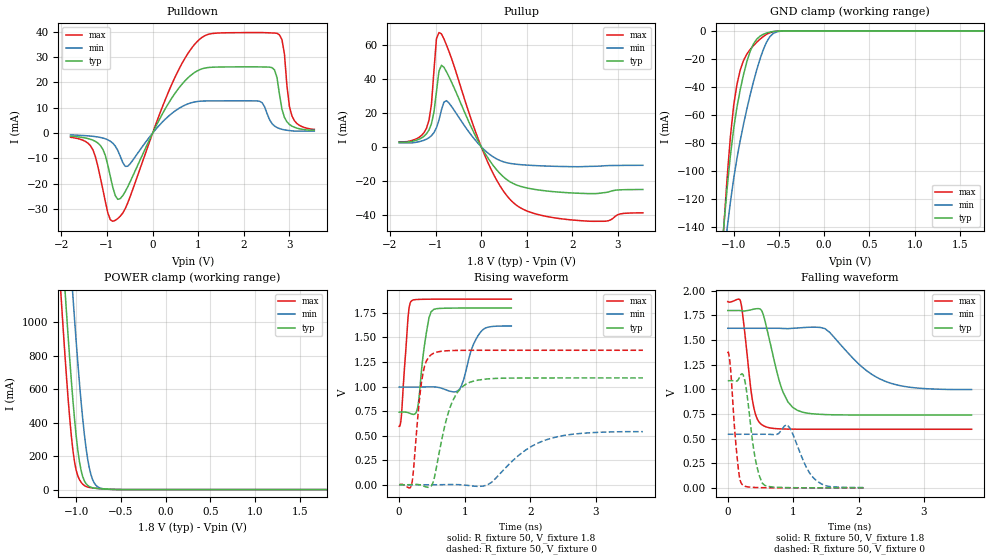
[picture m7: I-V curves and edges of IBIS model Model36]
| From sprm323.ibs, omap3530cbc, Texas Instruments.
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| Model based on original model for BQOMAPPROGIOCSHYFBPB_7LM
|   Sub model MODE10_PU_PD_OFF_1P8
[model]   Model36
|[Input Load]   PI
|[Output Drive] DS10
|Voltage   1.8V
|Mode   I/O
Model_type   I/O
Polarity   Non-Inverting
Enable   Active-Low
Vinl =  0.63
Vinh =  1.17
Cref =  15.0000pF
Rref =  100.0000M
Vref =  0V
Vmeas =  0.9
C_comp   0.8864943p   0.7714798p   1.034566p
[Model Spec]
Vinl   0.63   0.567   0.6615
Vinh   1.17   1.053   1.2285
[Temperature Range]   25   125   -40
[Voltage Range]   1.8   1.62   1.89
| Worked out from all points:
|   slope of the pulldown table from 0 to 0.27 V, typ, clamps not added: 28.9 ohm
|   slope of the pullup table from 0 to 0.27 V, typ, clamps not added: 24 ohm
|   GND clamp passes 1 mA (typ) near -0.61 V on its own axis
|   POWER clamp passes 1 mA (typ) near -0.56 V on its own axis
|   rising waveform, R_fixture 50, V_fixture 1.8: 20-80 % time 113ps typ, 178ps min, 78.6ps max; typ from 0.739 V to 1.8 V
|   rising waveform, R_fixture 50, V_fixture 0: 20-80 % time 249ps typ, 614ps min, 120ps max; typ from 0 V to 1.09 V
|   falling waveform, R_fixture 50, V_fixture 1.8: 20-80 % time 253ps typ, 609ps min, 137ps max; typ from 1.8 V to 0.739 V
|   falling waveform, R_fixture 50, V_fixture 0: 20-80 % time 137ps typ, 238ps min, 93.4ps max; typ from 1.09 V to 0 V
[POWER_clamp]
-1.8V     7.429A     8.065A     7.064A
-1.182V   1.663A     2.35A      1.259A
-1.164V   1.508A     2.193A     1.106A
-1.127V   1.206A     1.883A     813.2mA
-1.073V   782.1mA    1.435A     426.3mA
-1.036V   530.6mA    1.15A      232.4mA
-981.8mV  234.7mA    756.3mA    81.67mA
-909.1mV  52.8mA     331.4mA    24.39mA
-872.7mV  25.58mA    185.5mA    15.34mA
-818.2mV  11.18mA    61.99mA    9.987mA
-709.1mV  4.516mA    6.134mA    4.387mA
1.8V      470.6pA    2.239nA    626.3pA
[Pulldown]
-1.8V     -1.194mA   -708.4uA   -1.62mA
-1.364V   -2.427mA   -1.16mA    -4.962mA
-1.145V   -4.869mA   -1.705mA   -17.58mA
-818.2mV  -24.64mA   -5.097mA   -34.41mA
-545.5mV  -21.18mA   -13.06mA   -27.54mA
654.5mV   19.52mA    10.56mA    27.82mA
1.527V    26.09mA    12.74mA    39.54mA
2.345V    26.12mA    12.56mA    39.67mA
2.618V    25.84mA    3.762mA    39.51mA
2.782V    15.29mA    1.796mA    38.75mA
3.055V    2.769mA    903.4uA    6.806mA
3.545V    1.202mA    771.2uA    1.468mA
[Pullup]
-1.8V     2.751mA    2.282mA    2.931mA
-1.2V     7.642mA    4.475mA    10.93mA
-1.091V   13.62mA    6.537mA    25.15mA
-1.036V   20.45mA    8.342mA    44.84mA
-981.8mV  32.37mA    11.16mA    63.54mA
-927.3mV  44.36mA    15.62mA    67.08mA
-872.7mV  47.84mA    21.61mA    66.32mA
-763.6mV  44.16mA    27.09mA    59.89mA
54.55mV   -2.548mA   -1.463mA   -3.577mA
709.1mV   -21.68mA   -10.05mA   -32.93mA
2.127V    -27.28mA   -11.7mA    -43.28mA
3.545V    -25.07mA   -10.87mA   -38.77mA
[GND_clamp]
-1.8V     -794.1mA   -670.5mA   -980.8mA
-1.109V   -139.6mA   -162.5mA   -140mA
-1.073V   -112.7mA   -141.5mA   -105.3mA
-1.036V   -89.23mA   -122.4mA   -75.75mA
-1V       -69.83mA   -105.6mA   -53.36mA
-963.6mV  -54.49mA   -90.99mA   -38.21mA
-890.9mV  -31.19mA   -66.62mA   -21.14mA
-818.2mV  -14.71mA   -45.88mA   -13.31mA
-709.1mV  -3.87mA    -20.18mA   -5.973mA
-600mV    -903.1uA   -4.176mA   -1.354mA
-490.9mV  -116.3uA   -342.2uA   -105.5uA
1.764V    389.6pA    119.4nA    561.5pA
[Ramp]
dV/dt_f  0.6480462/0.2533436n  0.3821288/0.6207932n  0.7925844/0.1380049n
dV/dt_r  0.6684608/0.2495437n  0.3367728/0.6287017n  0.8410031/0.1201029n
R_load = 50
[Rising Waveform]
R_fixture = 50
V_fixture = 1.8
V_fixture_min = 1.62
V_fixture_max = 1.89
0s        739.2mV    994.5mV    594.8mV
32ps      740.1mV    994.5mV    680.8mV
136ps     734.3mV    994.5mV    1.706V
192ps     719.9mV    994.5mV    1.874V
280ps     776.5mV    994.5mV    1.886V
384ps     1.407V     995.8mV    1.889V
488ps     1.761V     996.9mV    1.889V
912ps     1.799V     965.1mV    1.89V
1.24ns    1.8V       1.552V     1.89V
1.712ns   1.8V       1.617V     1.89V
[Rising Waveform]
R_fixture = 50
V_fixture = 0
V_fixture_min = 0
V_fixture_max = 0
0s        320.1nV    197.1nV    708.6nV
184ps     1.066mV    3.334uV    -15.93mV
344ps     -7.515mV   -6.636uV   1.056V
416ps     -23.59mV   -106.3uV   1.26V
512ps     14.43mV    -92.34uV   1.334V
768ps     769.9mV    1.935mV    1.366V
1.016ns   1.023V     -4.316mV   1.369V
1.344ns   1.077V     -2.617mV   1.369V
2.272ns   1.087V     463.6mV    1.369V
3.72ns    1.088V     540.8mV    1.369V
[Falling Waveform]
R_fixture = 50
V_fixture = 1.8
V_fixture_min = 1.62
V_fixture_max = 1.89
0s        1.8V       1.62V      1.89V
192ps     1.8V       1.62V      1.902V
376ps     1.811V     1.62V      894mV
448ps     1.819V     1.62V      703.1mV
544ps     1.757V     1.62V      631.5mV
824ps     1.01V      1.619V     598.1mV
1.064ns   787.2mV    1.623V     595.4mV
1.488ns   744mV      1.616V     594.9mV
2.448ns   739.4mV    1.072V     594.8mV
3.728ns   739.3mV    997.8mV    594.8mV
[Falling Waveform]
R_fixture = 50
V_fixture = 0
V_fixture_min = 0
V_fixture_max = 0
0s        1.088V     544.1mV    1.369V
40ps      1.088V     544.1mV    1.229V
160ps     1.097V     544.1mV    203.4mV
216ps     1.159V     544.1mV    36.95mV
280ps     1.017V     544.1mV    13.38mV
424ps     284.7mV    544.1mV    3.882mV
528ps     47.25mV    544.2mV    1.831mV
904ps     2.687mV    641.6mV    141.8uV
1.352ns   303.6uV    76mV       9.618uV
2.088ns   19.76uV    3.318mV    856.9nV
